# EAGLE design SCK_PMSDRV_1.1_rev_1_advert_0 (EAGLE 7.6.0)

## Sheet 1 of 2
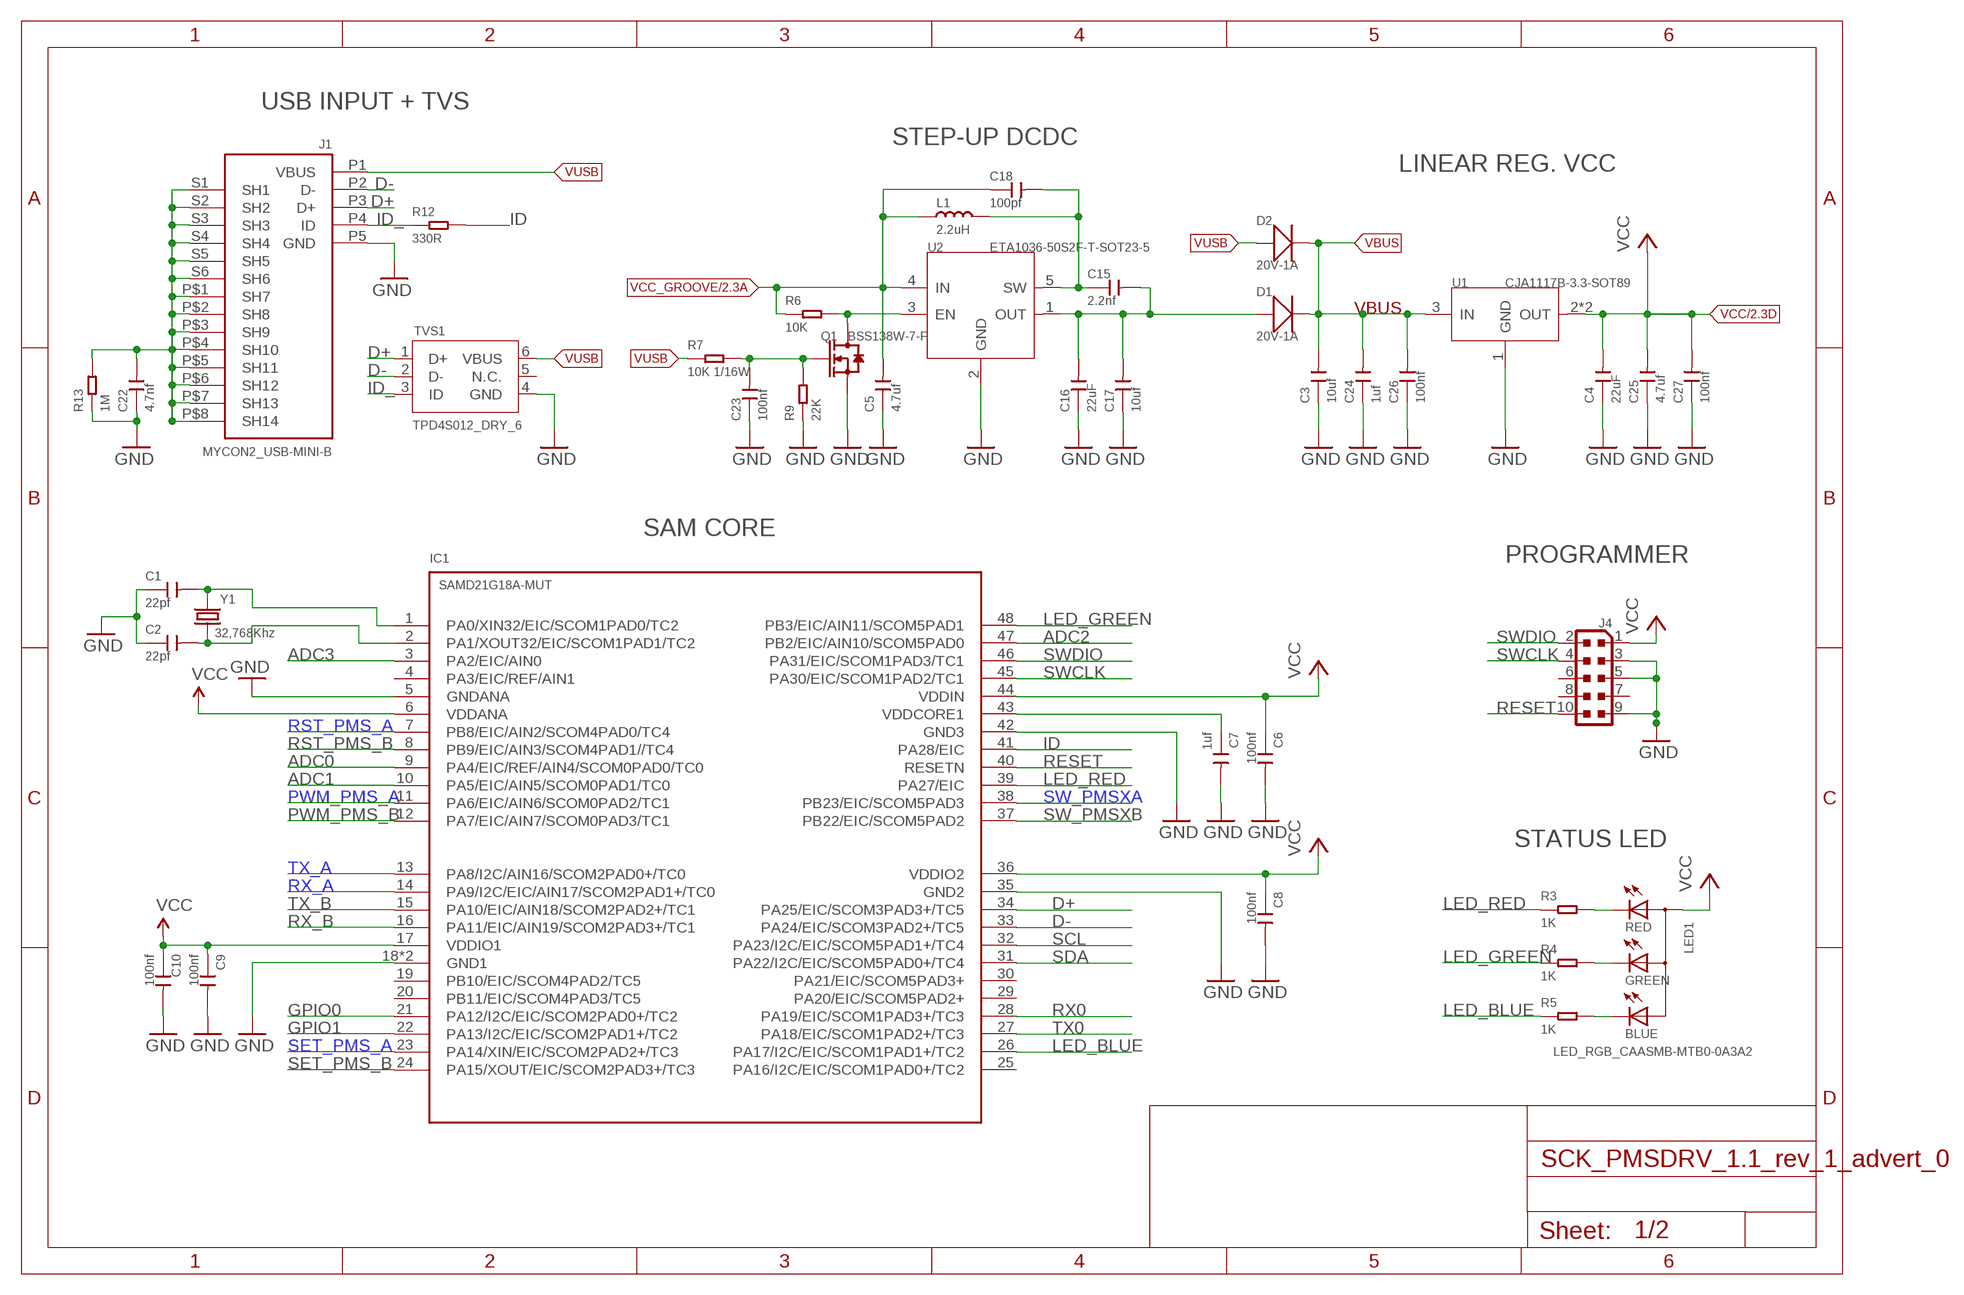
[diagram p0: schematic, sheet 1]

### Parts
C1  22pf  CERAMIC-22PF-50V-5%-NPO(0402)  [C0402]
C2  22pf  CERAMIC-22PF-50V-5%-NPO(0402)  [C0402]
C3  10uf  CERAMIC-10UF-25V-10%-X5R(1206)  [C1206]
C4  22uF  CERAMIC-22UF-16V-10%-X7R(1206)  [C1206]
C5  4.7uf  CERAMIC-4.7UF-25V-10%-X5R(0805)  [C0805]
C6  100nf  CERAMIC-100NF-50V-10%-X7R(0603)  [C0603]
C7  1uf  CERAMIC-1UF-25V-10%-X7R(0603)  [C0603]
C8  100nf  CERAMIC-100NF-50V-10%-X7R(0603)  [C0603]
C9  100nf  CERAMIC-100NF-50V-10%-X7R(0603)  [C0603]
C10  100nf  CERAMIC-100NF-50V-10%-X7R(0603)  [C0603]
C15  2.2nf  CERAMIC-2.2NF-50V-10%-X7R(0402)  [C0402]
C16  22uF  CERAMIC-22UF-16V-10%-X7R(1206)  [C1206]
C17  10uf  CERAMIC-10UF-25V-10%-X5R(1206)  [C1206]
C18  100pf  CERAMIC-100PF-50V-5%-NPO(0603)  [C0603]
C22  4.7nf  CERAMIC-4.7NF-50V-10%-X7R(0603)  [C0603]
C23  100nf  CERAMIC-100NF-50V-10%-X7R(0603)  [C0603]
C24  1uf  CERAMIC-1UF-25V-10%-X7R(0805)  [C0805]
C25  4.7uf  CERAMIC-4.7UF-25V-10%-X5R(0805)  [C0805]
C26  100nf  CERAMIC-100NF-50V-10%-X7R(0805)  [C0805]
C27  100nf  CERAMIC-100NF-50V-10%-X7R(0805)  [C0805]
D1  20V-1A  SMD-DIODE-SCHOTTKY-20V-1A(SOD-123)  [SOD-123]
D2  20V-1A  SMD-DIODE-SCHOTTKY-20V-1A(SOD-123)  [SOD-123]
IC1  SAMD21G18A-MUT  HANGAR_SAMD21G18A-MUT  [HANGAR_QFN48-7X7]
J1  MYCON2_USB-MINI-B  HANGAR_MYCON2_USB-MINI-B  [HANGAR_CON2_USB_MICRO_B_AT]
J4  HANGAR_PINHEAD_PINHD-2X5SMD  [HANGAR_2X05_SMD_1.27MM]
L1  2.2uH  SMD-INDUCTOR-10UH-20%-2.35A(2P-5X5X4MM)  [L5040S]
LED1  LED_RGB_CAASMB-MTB0-0A3A2  HANGAR_LED_RGB_CAASMB-MTB0-0A3A2  [HANGAR_P-LCC-4]
Q1  BSS138W-7-F  SMD-MOSFET-N-CH-50V-200MA-BSS138W-7-F(SOT-23)  [SOT-23]
R3  1K  SMD-RES-1K-5%-1/16W(0402)  [R0402]
R4  1K  SMD-RES-1K-5%-1/16W(0402)  [R0402]
R5  1K  SMD-RES-1K-5%-1/16W(0402)  [R0402]
R6  10K  SMD-RES-10K-1%-1/10W(0603)  [R0603]
R7  10K 1/16W  SMD-RES-10K-1%-1/16W(0402)  [R0402]
R9  22K  SMD-RES-22K-5%-1/10W(0603)  [R0603]
R12  330R  SMD-RES-330R-1%-1/10W(0603)  [R0603]
R13  1M  SMD-RES-1M-1%-1/10W(0603)  [R0603]
TVS1  TPD4S012_DRY_6  [DRY6]
U1  CJA1117B-3.3-SOT89  PMIC-CJA1117B-3.3(SOT-89)  [SOT-89]
U2  ETA1036-50S2F-T-SOT23-5  PMIC-ETA1036-50S2F-T(SOT23-5)  [SOT-23-5]
Y1  32,768Khz  0213_ABS07-32.768KHZ-T  [RESONATOR_EPSON_FC_145]

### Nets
ADC0: IC1.9(PA4/EIC/REF/AIN4/SCOM0PAD0/TC0) ; also sheet 2
ADC1: IC1.10(PA5/EIC/AIN5/SCOM0PAD1/TC0) ; also sheet 2
ADC2: IC1.47(PB2/EIC/AIN10/SCOM5PAD0) ; also sheet 2
ADC3: IC1.3(PA2/EIC/AIN0) ; also sheet 2
D+: IC1.34(PA25/EIC/SCOM3PAD3+/TC5) J1.P3(D+) TVS1.1(D+)
D-: IC1.33(PA24/EIC/SCOM3PAD2+/TC5) J1.P2(D-) TVS1.2(D-)
GND: C1.1 C2.1 C3.1 C4.1 C5.1 C6.2 C7.2 C8.2 C9.2 C10.2 C16.1 C17.1 C22.1 C23.1 C24.1 C25.1 C26.1 C27.1 IC1.5(GNDANA) IC1.18(GND1) IC1.35(GND2) IC1.42(GND3) IC1.TP(GND1) J1.P5(GND) J4.3 J4.5 J4.9 Q1.2(S) R9.1 R13.1 TVS1.4(GND) U1.1(GND) U2.2(GND) ; also sheet 2
GPIO0: IC1.21(PA12/I2C/EIC/SCOM2PAD0+/TC2) ; also sheet 2
GPIO1: IC1.22(PA13/I2C/EIC/SCOM2PAD1+/TC2) ; also sheet 2
ID: IC1.41(PA28/EIC) R12.2
ID_: J1.P4(ID) R12.1 TVS1.3(ID)
LED_BLUE: IC1.26(PA17/I2C/EIC/SCOM1PAD1+/TC2) R5.1
LED_GREEN: IC1.48(PB3/EIC/AIN11/SCOM5PAD1) R4.1
LED_RED: IC1.39(PA27/EIC) R3.1
N$1: LED1.4(RED) R3.2
N$2: LED1.3(GREEN) R4.2
N$3: LED1.2(BLUE) R5.2
N$4: C7.1 IC1.43(VDDCORE1)
N$6: Q1.3(D) R6.2 U2.3(EN)
N$7: C23.2 Q1.1(G) R7.2 R9.2
N$8: C15.1 C18.2 L1.2 U2.5(SW)
PA00_XIN32: C1.2 IC1.1(PA0/XIN32/EIC/SCOM1PAD0/TC2) Y1.P$2
PA01_XOUT32: C2.2 IC1.2(PA1/XOUT32/EIC/SCOM1PAD1/TC2) Y1.P$1
PWM_PMS_A: IC1.11(PA6/EIC/AIN6/SCOM0PAD2/TC1) ; also sheet 2
PWM_PMS_B: IC1.12(PA7/EIC/AIN7/SCOM0PAD3/TC1) ; also sheet 2
RESET: IC1.40(RESETN) J4.10
RST_PMS_A: IC1.7(PB8/EIC/AIN2/SCOM4PAD0/TC4) ; also sheet 2
RST_PMS_B: IC1.8(PB9/EIC/AIN3/SCOM4PAD1//TC4) ; also sheet 2
RX0: IC1.28(PA19/EIC/SCOM1PAD3+/TC3) ; also sheet 2
RX_A: IC1.14(PA9/I2C/EIC/AIN17/SCOM2PAD1+/TC0) ; also sheet 2
RX_B: IC1.16(PA11/EIC/AIN19/SCOM2PAD3+/TC1) ; also sheet 2
SCL: IC1.32(PA23/I2C/EIC/SCOM5PAD1+/TC4) ; also sheet 2
SDA: IC1.31(PA22/I2C/EIC/SCOM5PAD0+/TC4) ; also sheet 2
SET_PMS_A: IC1.23(PA14/XIN/EIC/SCOM2PAD2+/TC3) ; also sheet 2
SET_PMS_B: IC1.24(PA15/XOUT/EIC/SCOM2PAD3+/TC3) ; also sheet 2
SHIELD: C22.2 J1.P$1(SH7) J1.P$2(SH8) J1.P$3(SH9) J1.P$4(SH10) J1.P$5(SH11) J1.P$6(SH12) J1.P$7(SH13) J1.P$8(SH14) J1.S1(SH1) J1.S2(SH2) J1.S3(SH3) J1.S4(SH4) J1.S5(SH5) J1.S6(SH6) R13.2
SW_PMSXA: IC1.38(PB23/EIC/SCOM5PAD3) ; also sheet 2
SW_PMSXB: IC1.37(PB22/EIC/SCOM5PAD2) ; also sheet 2
SWCLK: IC1.45(PA30/EIC/SCOM1PAD2/TC1) J4.4
SWDIO: IC1.46(PA31/EIC/SCOM1PAD3/TC1) J4.2
TX0: IC1.27(PA18/EIC/SCOM1PAD2+/TC3) ; also sheet 2
TX_A: IC1.13(PA8/I2C/AIN16/SCOM2PAD0+/TC0) ; also sheet 2
TX_B: IC1.15(PA10/EIC/AIN18/SCOM2PAD2+/TC1) ; also sheet 2
VBUS: C3.2 C24.2 C26.2 D1.- D2.- U1.3(IN) ; also sheet 2
VCC [usbvcc]: C4.2 C6.1 C8.1 C9.1 C10.1 C25.2 C27.2 IC1.6(VDDANA) IC1.17(VDDIO1) IC1.36(VDDIO2) IC1.44(VDDIN) J4.1 LED1.1(A) U1.2(OUT) U1.4(OUT) ; also sheet 2
VCC_GROOVE: C5.2 C18.1 L1.1 R6.1 U2.4(IN) ; also sheet 2
VO_DCDC: C15.2 C16.2 C17.2 D1.+ U2.1(OUT)
VUSB: D2.+ J1.P1(VBUS) R7.1 TVS1.6(VBUS)
Unconnected: IC1.4(PA3/EIC/REF/AIN1) IC1.19(PB10/EIC/SCOM4PAD2/TC5) IC1.20(PB11/EIC/SCOM4PAD3/TC5) IC1.25(PA16/I2C/EIC/SCOM1PAD0+/TC2) IC1.29(PA20/EIC/SCOM5PAD2+) IC1.30(PA21/EIC/SCOM5PAD3+) J4.6 J4.7 J4.8 TVS1.5(N.C.)

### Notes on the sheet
- USB INPUT + TVS
- STEP-UP DCDC
- LINEAR REG. VCC
- SAM CORE
- PROGRAMMER
- STATUS LED

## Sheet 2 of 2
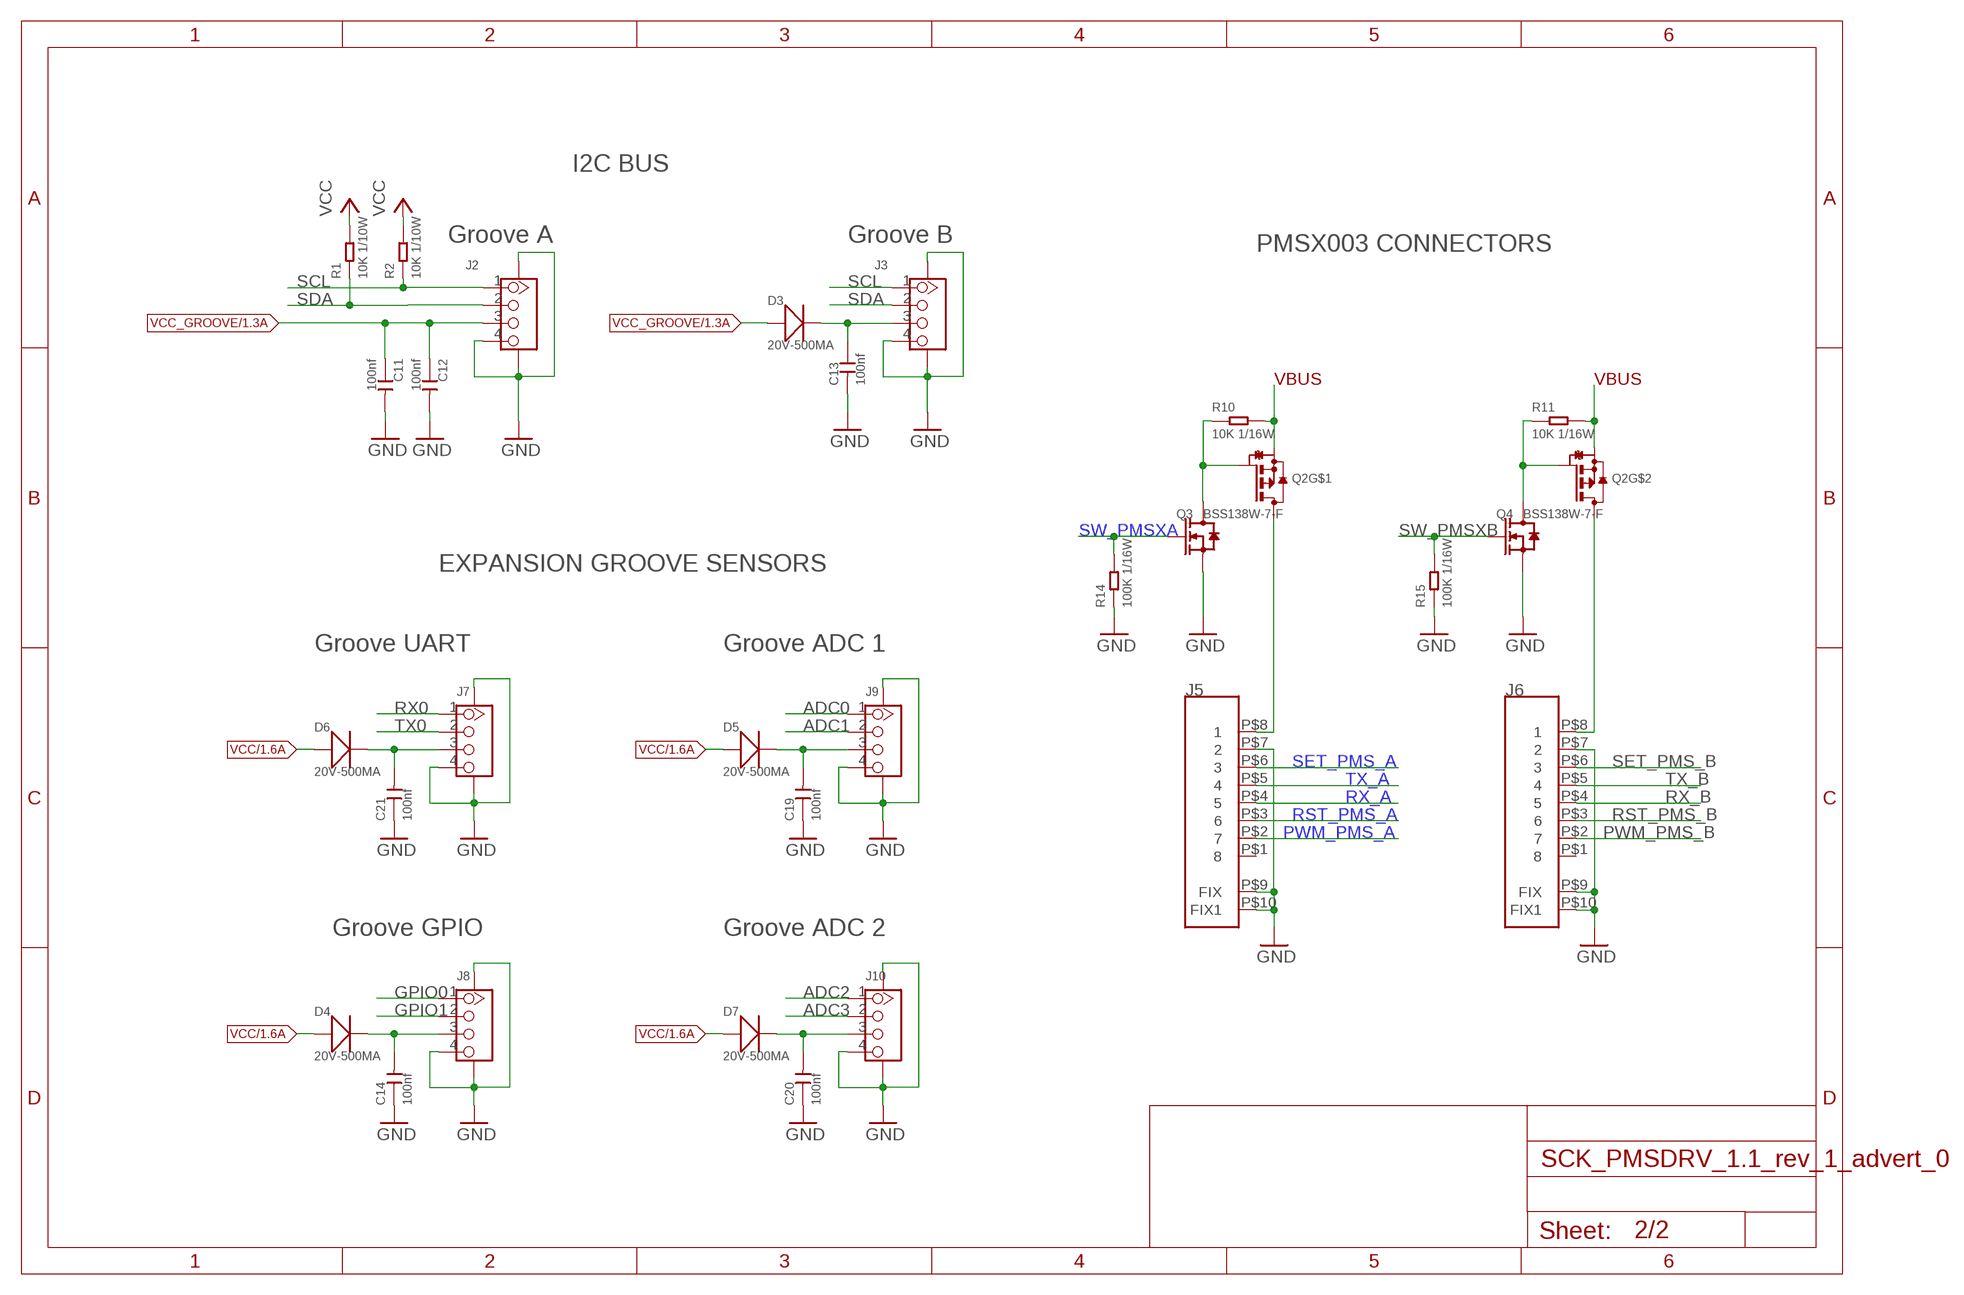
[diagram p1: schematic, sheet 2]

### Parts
C11  100nf  CERAMIC-100NF-50V-10%-X7R(0603)  [C0603]
C12  100nf  CERAMIC-100NF-50V-10%-X7R(0603)  [C0603]
C13  100nf  CERAMIC-100NF-50V-10%-X7R(0603)  [C0603]
C14  100nf  CERAMIC-100NF-50V-10%-X7R(0603)  [C0603]
C19  100nf  CERAMIC-100NF-50V-10%-X7R(0603)  [C0603]
C20  100nf  CERAMIC-100NF-50V-10%-X7R(0603)  [C0603]
C21  100nf  CERAMIC-100NF-50V-10%-X7R(0603)  [C0603]
D3  20V-500MA  SMD-DIODE-SCHOTTKY-20V-500MA(SOD-123)P  [SOD-123]
D4  20V-500MA  SMD-DIODE-SCHOTTKY-20V-500MA(SOD-123)P  [SOD-123]
D5  20V-500MA  SMD-DIODE-SCHOTTKY-20V-500MA(SOD-123)P  [SOD-123]
D6  20V-500MA  SMD-DIODE-SCHOTTKY-20V-500MA(SOD-123)P  [SOD-123]
D7  20V-500MA  SMD-DIODE-SCHOTTKY-20V-500MA(SOD-123)P  [SOD-123]
J2  CONNECTOR-NEW_GROVE-CONNECTOR-SMD90D  [CONNECTOR-NEW_HW4-SMD-2.0-90D]
J3  CONNECTOR-NEW_GROVE-CONNECTOR-SMD90D  [CONNECTOR-NEW_HW4-SMD-2.0-90D]
J5  MOLEX_53398-0871_8PIN  [MOLEX_PICOBLADE_8PIN]
J6  MOLEX_53398-0871_8PIN  [MOLEX_PICOBLADE_8PIN]
J7  CONNECTOR-NEW_GROVE-CONNECTOR-SMD90D  [CONNECTOR-NEW_HW4-SMD-2.0-90D]
J8  CONNECTOR-NEW_GROVE-CONNECTOR-SMD90D  [CONNECTOR-NEW_HW4-SMD-2.0-90D]
J9  CONNECTOR-NEW_GROVE-CONNECTOR-SMD90D  [CONNECTOR-NEW_HW4-SMD-2.0-90D]
J10  CONNECTOR-NEW_GROVE-CONNECTOR-SMD90D  [CONNECTOR-NEW_HW4-SMD-2.0-90D]
Q2  MOSFETP_BOTH  [HANGAR_POWERPAKSC70-6L]
Q3  BSS138W-7-F  SMD-MOSFET-N-CH-50V-200MA-BSS138W-7-F(SOT-23)  [SOT-23]
Q4  BSS138W-7-F  SMD-MOSFET-N-CH-50V-200MA-BSS138W-7-F(SOT-23)  [SOT-23]
R1  10K 1/10W  SMD-RES-10K-5%-1/10W(0603)  [R0603]
R2  10K 1/10W  SMD-RES-10K-5%-1/10W(0603)  [R0603]
R10  10K 1/16W  SMD-RES-10K-1%-1/16W(0402)  [R0402]
R11  10K 1/16W  SMD-RES-10K-1%-1/16W(0402)  [R0402]
R14  100K 1/16W  SMD-RES-100K-5%-1/16W(0402)  [R0402]
R15  100K 1/16W  SMD-RES-100K-5%-1/16W(0402)  [R0402]

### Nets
ADC0: J9.1 ; also sheet 1
ADC1: J9.2 ; also sheet 1
ADC2: J10.1 ; also sheet 1
ADC3: J10.2 ; also sheet 1
GND: C11.2 C12.2 C13.2 C14.1 C19.1 C20.1 C21.1 J2.4 J2.SS1 J2.SS2 J3.4 J3.SS1 J3.SS2 J5.P$7 J5.P$9(FIX) J5.P$10(FIX1) J6.P$7 J6.P$9(FIX) J6.P$10(FIX1) J7.4 J7.SS1 J7.SS2 J8.4 J8.SS1 J8.SS2 J9.4 J9.SS1 J9.SS2 J10.4 J10.SS1 J10.SS2 Q3.2(S) Q4.2(S) R14.1 R15.1 ; also sheet 1
GPIO0: J8.1 ; also sheet 1
GPIO1: J8.2 ; also sheet 1
N$9: J5.P$8 Q2.6(D) Q2.TP1(D)
N$10: J6.P$8 Q2.3(D) Q2.TP2(D)
N$12: C14.2 D4.- J8.3
N$13: C19.2 D5.- J9.3
N$14: C21.2 D6.- J7.3
N$15: C20.2 D7.- J10.3
N$16: C13.1 D3.- J3.3
PWM_PMS_A: J5.P$2 ; also sheet 1
PWM_PMS_B: J6.P$2 ; also sheet 1
RST_PMS_A: J5.P$3 ; also sheet 1
RST_PMS_B: J6.P$3 ; also sheet 1
RX0: J7.1 ; also sheet 1
RX_A: J5.P$4 ; also sheet 1
RX_B: J6.P$4 ; also sheet 1
SCL: J2.1 J3.1 R2.1 ; also sheet 1
SDA: J2.2 J3.2 R1.1 ; also sheet 1
SET_PMS_A: J5.P$6 ; also sheet 1
SET_PMS_B: J6.P$6 ; also sheet 1
SW_PMSXA: Q3.1(G) R14.2 ; also sheet 1
SW_PMSXA_NEG: Q2.2(G) Q3.3(D) R10.1
SW_PMSXB: Q4.1(G) R15.2 ; also sheet 1
SW_PMSXB_NEG: Q2.5(G) Q4.3(D) R11.1
TX0: J7.2 ; also sheet 1
TX_A: J5.P$5 ; also sheet 1
TX_B: J6.P$5 ; also sheet 1
VBUS: Q2.1(S) Q2.4(S) R10.2 R11.2 ; also sheet 1
VCC [usbvcc]: D4.+ D5.+ D6.+ D7.+ R1.2 R2.2 ; also sheet 1
VCC_GROOVE: C11.1 C12.1 D3.+ J2.3 ; also sheet 1
Unconnected: J5.P$1 J6.P$1

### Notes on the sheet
- I2C BUS
- Groove A | Groove B
- PMSX003 CONNECTORS
- EXPANSION GROOVE SENSORS
- Groove UART | Groove ADC 1
- Groove GPIO | Groove ADC 2

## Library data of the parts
C1 C2 = Seeed-Capacitor:CERAMIC-22PF-50V-5%-NPO(0402): 302010018; MPN: CC0402JRNPO9BN220
C3 C17 = Seeed-Capacitor:CERAMIC-10UF-25V-10%-X5R(1206): 302010181; MPN: CC1206KKX5R8BB106
C4 C16 = Seeed-Capacitor:CERAMIC-22UF-16V-10%-X7R(1206): 302010182
C5 C25 = Seeed-Capacitor:CERAMIC-4.7UF-25V-10%-X5R(0805): 302010146; MPN: CC0805KKX5R8BB475
C6 C8-C14 C19-C21 C23 = Seeed-Capacitor:CERAMIC-100NF-50V-10%-X7R(0603): 302010138; MPN: CC0603KRX7R9BB104
C7 = Seeed-Capacitor:CERAMIC-1UF-25V-10%-X7R(0603): 302010139; MPN: CC0603KRX7R8BB105
C15 = Seeed-Capacitor:CERAMIC-2.2NF-50V-10%-X7R(0402): 302010022; MPN: CC0402KRX7R9BB222
C18 = Seeed-Capacitor:CERAMIC-100PF-50V-5%-NPO(0603): 302010076; MPN: CC0603JRNPO9BN101
C22 = Seeed-Capacitor:CERAMIC-4.7NF-50V-10%-X7R(0603): 302010144; MPN: CC0603KRX7R9BB472
C24 = Seeed-Capacitor:CERAMIC-1UF-25V-10%-X7R(0805): 302010179; MPN: CC0805KKX7R8BB105
C26 C27 = Seeed-Capacitor:CERAMIC-100NF-50V-10%-X7R(0805): 302010165; MPN: CC0805KRX7R9BB104
D1 D2 = Seeed-OPL-Diode:SMD-DIODE-SCHOTTKY-20V-1A(SOD-123): 304020034; MPN: B5819W
D3-D7 = Seeed-Diode:SMD-DIODE-SCHOTTKY-20V-500MA(SOD-123)P: 304020028; MPN: MBR0520LT1G
IC1 = SCK_BASE_BOARD_v1.6:HANGAR_SAMD21G18A-: Atmel D21 32bit ARM Cortex-M0 microcontroller - 48 PIN TQFP 256KB flash memory + 32KB SRAM
J1 = SCK_BASE_BOARD_v1.6:HANGAR_MYCON2_USB-MINI-B
J2 J3 J7-J10 = SCK_BASE_BOARD_v1.6:CONNECTOR-NEW_GROVE-CONNECTOR-SMD: 4P-SMD-2.0:320110030;4P-SMD-2.0-90D:320110032
J4 = SCK_BASE_BOARD_v1.6:HANGAR_PINHEAD_PINHD-2X5: PIN HEADER
J5 J6 = SCK_BASE_BOARD_v1.6:MOLEX_53398-0871_8PIN
L1 = Seeed-Inductor:SMD-INDUCTOR-10UH-20%-2.35A(2P-5X5X4MM): 303010147
LED1 = SCK_BASE_BOARD_v1.6:HANGAR_LED_RGB_CA: PLCC-4 RGB LED
Q1 Q3 Q4 = Seeed-Transistor:SMD-MOSFET-N-CH-50V-200MA-BSS138W-7-F(SOT-23): 305030000; MPN: BSS138W-7-F
Q2 = SCK_BASE_BOARD_v1.6:MOSFETP_BOTH
R1 R2 = Seeed-Resistor:SMD-RES-10K-5%-1/10W(0603): 301010293; MPN: RC0603JR-0710KL
R3-R5 = Seeed-Resistor:SMD-RES-1K-5%-1/16W(0402): 301010006; MPN: RC0402JR-071KL
R6 = Seeed-Resistor:SMD-RES-10K-1%-1/10W(0603): 301010299; MPN: RC0603FR-0710KL
R7 R10 R11 = Seeed-Resistor:SMD-RES-10K-1%-1/16W(0402): 301010047; MPN: RC0402FR-0710KL
R9 = Seeed-Resistor:SMD-RES-22K-5%-1/10W(0603): 301010132; MPN: RC0603JR-0722KL
R12 = Seeed-Resistor:SMD-RES-330R-1%-1/10W(0603): 301010300; MPN: RC0603FR-07330RL
R13 = Seeed-Resistor:SMD-RES-1M-1%-1/10W(0603): 301010151; MPN: RC0603FR-071ML
R14 R15 = Seeed-Resistor:SMD-RES-100K-5%-1/16W(0402): 301010033; MPN: RC0402JR-07100KL
TVS1 = fabhack:TPD4S012_DRY_6
U1 = Seeed-IC:PMIC-CJA1117B-3.3(SOT-89): 310030095; MPN: CJA1117B-3.3
U2 = Seeed-IC:PMIC-ETA1036-50S2F-T(SOT23-5): 310030153; MPN: ETA1036-50S2F-T
Y1 = Cristalli:0213_ABS07-32.768KHZ-T: 32,768KHz - SMD; MONTHLY_USAGE: _____; PART_NUMBER: ABS07-32.768KHZ-T; PRICE: _____; SUPPLIER: _____; TYPE: Cristalli; VALUE: 32,768Khz_SMD

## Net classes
0 Default: width 0.203 mm
1 power: width 1 mm, drill 0.6 mm, clearance 0.203 mm
2 gnd: width 0.254 mm, drill 0.6 mm, clearance 0.203 mm
3 usbvcc: width 0.254 mm, drill 0.6 mm, clearance 0.203 mm
4 aref: width 0.254 mm, drill 0.6 mm, clearance 0.203 mm

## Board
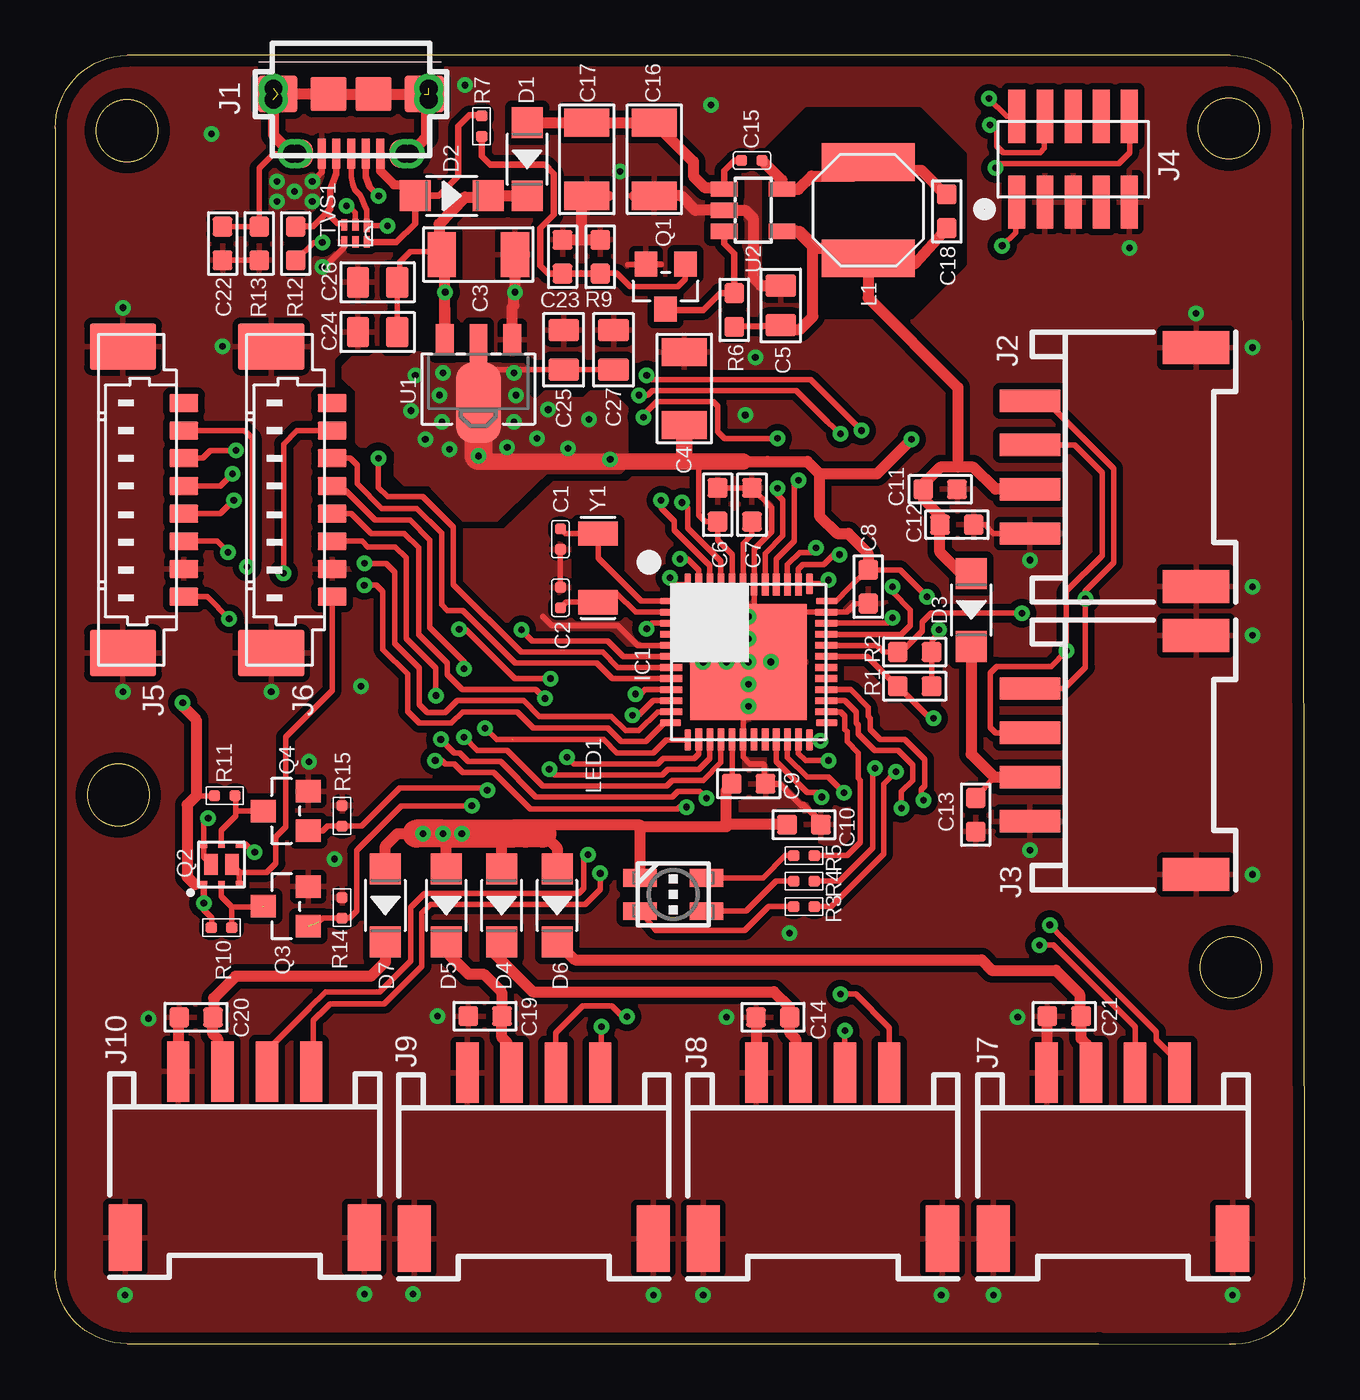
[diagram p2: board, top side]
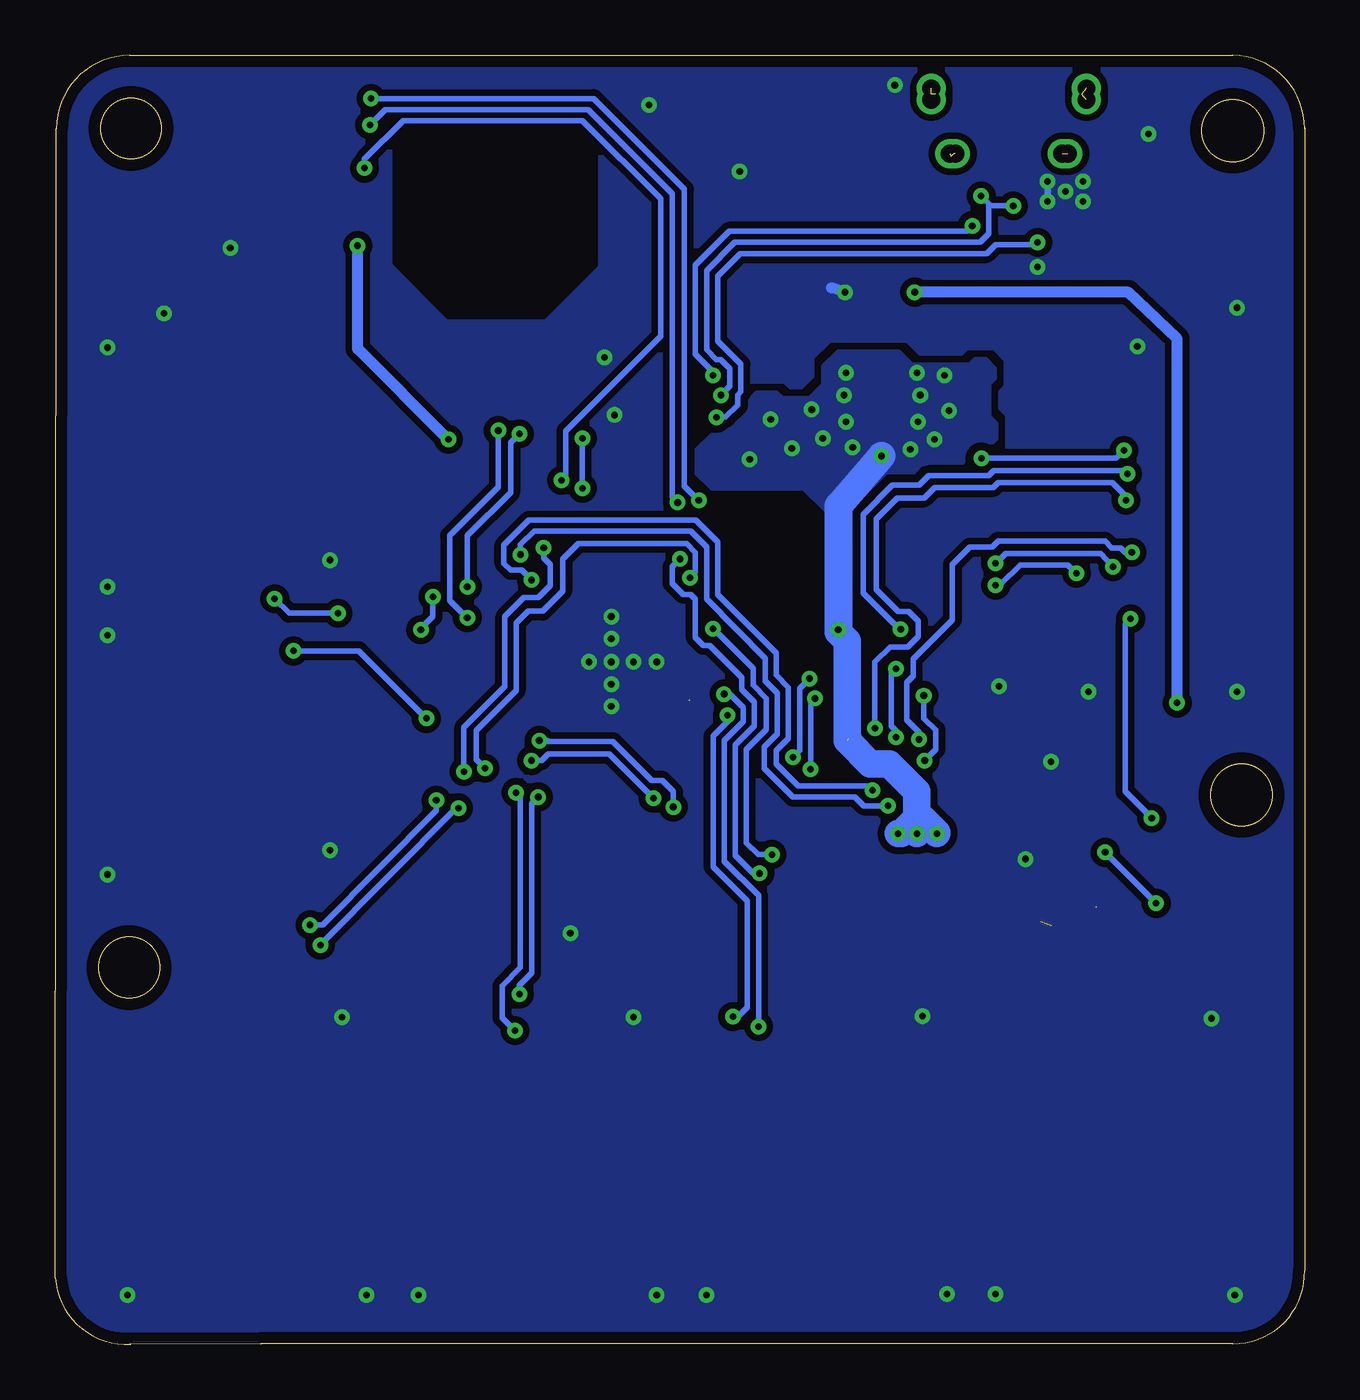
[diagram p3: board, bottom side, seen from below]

Size 56.4 x 58.21 mm. Coordinates in mm from the lower left corner, seen from the top.
Outline: 53,0 arc90 56.4,3.01 56.35,54.91 arc90 53.05,58.21 3.24,58.21 arc90 0,54.91
Outline: 0.9,0.98 arc45 3.24,0.02 47.11,0.02 arc90 47.12,0.02 53.03,0
Outline: 0.9,0.98 arc-45 0,3.32 0,54.94
Outline: circle at 53.07,17.01 radius 1.38
Outline: circle at 52.98,54.91 radius 1.38
Outline: circle at 3.24,54.81 radius 1.4
Outline: circle at 2.85,24.81 radius 1.4
Copper layers (1*16): Top 0.035mm / dielectric 1.5mm / Bottom 0.035mm
Design rules "default *": minimum track width 0.2mm, minimum drill 0.3mm, track to track 0.2mm, track to pad 0.2mm, pad to pad 0.2mm, via to via 0.2mm, smd to smd 0.2mm, copper to edge 20mil, drill to drill 0.6mm, minimum pad ring 10mil, minimum via ring 0.2mm, stop-mask expansion 2mil, vias tented up to drill 24mil, thermal gap 10mil

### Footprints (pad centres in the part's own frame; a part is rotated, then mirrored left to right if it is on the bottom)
C0402 = smd 0.5 x 0.5: 1 0,0.463; 2 0,-0.463
C1206 = smd 1.27 x 2.032: 1 -1.651,0; 2 1.651,0
C0805 = smd 1.397 x 1.016: 1 0,0.889; 2 0,-0.889
C0603 = smd 0.889 x 0.889: 1 0,0.762; 2 0,-0.762
SOD-123 = smd 1.397 x 1.397: + -1.651,0; - 1.651,0
HANGAR_QFN48-7X7 = smd 0.95 x 0.3: 1 -3.525,2.75; 12 -3.525,-2.75; 25 3.525,-2.75; 36 3.525,2.75 | smd 1 x 0.3: 2 -3.5,2.25; 3 -3.5,1.75; 4 -3.5,1.25; 5 -3.5,0.75; 6 -3.5,0.25; 7 -3.5,-0.25; 8 -3.5,-0.75; 9 -3.5,-1.25; 10 -3.5,-1.75; 11 -3.5,-2.25; 26 3.5,-2.25; 27 3.5,-1.75; 28 3.5,-1.25; 29 3.5,-0.75; 30 3.5,-0.25; 31 3.5,0.25; 32 3.5,0.75; 33 3.5,1.25; 34 3.5,1.75; 35 3.5,2.25 | smd 0.3 x 0.95: 13 -2.75,-3.525; 24 2.75,-3.525; 37 2.75,3.525; 48 -2.75,3.525 | smd 0.3 x 1: 14 -2.25,-3.5; 15 -1.75,-3.5; 16 -1.25,-3.5; 17 -0.75,-3.5; 18 -0.25,-3.5; 19 0.25,-3.5; 20 0.75,-3.5; 21 1.25,-3.5; 22 1.75,-3.5; 23 2.25,-3.5; 38 2.25,3.5; 39 1.75,3.5; 40 1.25,3.5; 41 0.75,3.5; 42 0.25,3.5; 43 -0.25,3.5; 44 -0.75,3.5; 45 -1.25,3.5; 46 -1.75,3.5; 47 -2.25,3.5 | smd 5.25 x 5.25: TP 0,0
HANGAR_CON2_USB_MICRO_B_AT = smd 0.406 x 1.346: P1 -1.321,2.692; P2 -0.66,2.692; P3 0,2.692; P4 0.66,2.692; P5 1.321,2.692 | drill 0.8 pad 1.27: P$1 -2.666,2.692 | drill 0.8 pad 1.245: P$2 -2.412,2.692; P$7 2.412,2.692; P$8 2.666,2.692 | drill 0.8 pad 1.143: P$3 -3.505,-0.254; P$4 -3.505,0.254; P$5 3.505,0.254; P$6 3.505,-0.254 | smd 1.778 x 1.651: S1 -3.302,0; S2 3.302,0 | smd 1.524 x 1.27: S3 -2.489,2.692; S4 2.489,2.692 | smd 1.626 x 1.524: S5 -1.016,0; S6 1.016,0
CONNECTOR-NEW_HW4-SMD-2.0-90D = smd 1.01 x 2.74: 1 -3,-0.1; 2 -1,-0.1; 3 1,-0.1; 4 3,-0.1 | smd 1.5 x 3: SS1 -5.4,7.4; SS2 5.4,7.4
HANGAR_2X05_SMD_1.27MM = smd 0.76 x 2.4: 1 -2.54,-1.94; 2 -2.54,1.94; 3 -1.27,-1.94; 4 -1.27,1.94; 5 0,-1.94; 6 0,1.94; 7 1.27,-1.94; 8 1.27,1.94; 9 2.54,-1.94; 10 2.54,1.94
MOLEX_PICOBLADE_8PIN = smd 0.8 x 1.3: P$1 0,0; P$2 1.25,0; P$3 2.5,0; P$4 3.75,0; P$5 5,0; P$6 6.25,0; P$7 7.5,0; P$8 8.75,0 | smd 2.1 x 3: P$9 -2.55,-2.75; P$10 11.3,-2.75
L5040S = smd 4.2 x 1.7: 1 0,2.175; 2 0,-2.175
HANGAR_P-LCC-4 = smd 0.8 x 1.5: 1 -0.75,-1.5; 2 -0.75,1.5; 3 0.75,1.5; 4 0.75,-1.5
SOT-23 = smd 1.016 x 1.143: 1 -0.889,-1.016; 2 0.889,-1.016; 3 0,1.016
HANGAR_POWERPAKSC70-6L = smd 0.3 x 0.325: 1 -0.8,-0.912; 2 0,-0.912; 3 0.8,-0.912; 4 0.8,0.912; 5 0,0.912; 6 -0.8,0.912 | smd 0.613 x 0.95: TP1 -0.467,0; TP2 0.467,0
R0603 = smd 0.889 x 0.889: 1 0,0.762; 2 0,-0.762
R0402 = smd 0.5 x 0.5: 1 0,0.463; 2 0,-0.463
DRY6 = smd 0.559 x 0.305: 1 -0.356,0.508 | smd 0.508 x 0.305: 2 -0.381,0; 3 -0.381,-0.508; 4 0.381,-0.508; 5 0.381,0; 6 0.381,0.508
SOT-89 = smd 0.8 x 1.4: 1 -1.524,-1.905; 3 1.524,-1.905 | smd 0.8 x 1.9: 2 0,-1.651 | smd 2.032 x 3.65: 4 0,0.94
SOT-23-5 = smd 0.69 x 1.2: 1 -0.95,-1.3; 2 0,-1.3; 3 0.95,-1.3; 4 0.95,1.3; 5 -0.95,1.3
RESONATOR_EPSON_FC_145 = smd 1.1 x 1.8: P$1 -1.55,0; P$2 1.55,0

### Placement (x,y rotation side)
C1  22.8,36.36 180 top
C2  22.8,33.71 0 top
C3  19.1,49.21 180 top
C4  28.4,43.16 270 top
C5  32.75,46.91 0 top
C6  29.9,37.91 180 top
C7  31.45,37.91 180 top
C8  36.7,34.21 0 top
C9  31.3,25.31 90 top
C10  33.8,23.46 90 top
C11  39.95,38.61 90 top
C12  40.7,37.01 90 top
C13  41.55,23.91 0 top
C14  32.4,14.76 90 top
C15  31.45,53.46 270 top
C16  27.05,53.51 90 top
C17  24,53.51 90 top
C18  40.25,51.16 180 top
C19  19.4,14.81 90 top
C20  6.35,14.76 90 top
C21  45.55,14.81 90 top
C22  7.55,49.71 180 top
C23  22.9,49.11 0 top
C24  14.55,45.71 90 top
C25  22.95,44.91 0 top
C26  14.55,47.96 90 top
C27  25.2,44.91 0 top
D1  21.3,53.51 270 top
D2  17.9,51.86 0 top
D3  41.35,33.16 270 top
D4  20.15,19.81 270 top
D5  17.65,19.81 270 top
D6  22.65,19.81 270 top
D7  14.9,19.81 270 top
IC1  31.3,30.81 0 top
J1  13.35,56.46 180 top
J2  44.1,39.61 270 top
J3  44.1,26.61 270 top
J4  45.95,53.51 0 top
J5  5.8,42.51 270 top
J6  12.5,42.51 270 top
J7  47.75,12.16 180 top
J8  34.65,12.16 180 top
J9  21.6,12.16 180 top
J10  8.55,12.21 180 top
L1  36.7,51.21 180 top
LED1  27.9,20.31 270 top
Q1  27.55,47.76 180 top
Q2  7.5,21.66 0 top
Q3  10.4,19.78 90 top
Q4  10.4,24.08 90 top
R1  38.8,29.71 90 top
R2  38.8,31.26 90 top
R3  33.8,19.76 270 top
R4  33.8,20.91 270 top
R5  33.8,22.06 270 top
R6  30.65,46.71 180 top
R7  19.25,55.01 0 top
R9  24.6,49.11 0 top
R10  7.5,18.81 270 top
R11  7.65,24.76 270 top
R12  10.85,49.71 0 top
R13  9.2,49.71 180 top
R14  12.95,19.71 0 top
R15  12.95,23.86 0 top
TVS1  13.55,50.16 270 top
U1  19.1,43.46 180 top
U2  31.5,51.21 270 top
Y1  24.5,35.06 90 top

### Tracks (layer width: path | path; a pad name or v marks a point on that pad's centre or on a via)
ADC0  (via drill 0.3)
  Top 0.25: v24.65,14.35 24.65,12.31 J9.1 | IC1.9 26.6,29.56 26.45,29.36 v26.2,29.36
  Bottom 0.25: v24.65,14.35 24.65,20.26 26.2,21.81 26.2,27.26 25.35,28.11 25.35,28.76 25.95,29.36 v26.2,29.36
ADC1  (via drill 0.3)  (1 unrouted)
  Top 0.25: J9.2 22.6,14.06 23.81,15.27 25.12,15.27 25.6,14.8 v25.81,14.8 | 27.75,29.06 27,29.06 26.35,28.41 v26.05,28.41
  Bottom 0.25: v26.05,28.41 26.05,28.11 26.7,27.46 26.7,21.56 25.15,20.01 25.15,15.21 25.61,14.75 25.82,14.79 v25.81,14.8
ADC2  (via drill 0.3)
  Top 0.25: IC1.47 29.05,34.97 28.56,35.46 v28.2,35.46 | J10.1 11.65,12.41 11.65,14.62 11.94,14.91 11.94,14.9 12.4,15.36 14.85,15.36 16.55,17.06 16.55,19.47 16.94,19.86 23.92,19.86 24.6,20.54 v24.6,21.26
  Bottom 0.25: v24.6,21.26 24.9,21.26 25.7,22.06 25.7,27.06 24.85,27.91 24.85,29.01 25.4,29.56 25.4,30.11 26.85,31.56 27.15,31.56 27.5,31.91 27.5,33.65 27.71,33.86 28.05,33.86 28.55,34.36 28.55,35.11 v28.2,35.46
ADC3  (via drill 0.3)
  Top 0.25: J10.2 9.55,13.25 11.46,15.16 11.46,15.18 12.2,15.91 14.65,15.91 16.05,17.31 16.05,19.73 16.68,20.36 23.63,20.36 23.85,20.59 23.85,21.91 v24.05,22.11 | IC1.3 26.95,32.56 v26.7,32.31
  Bottom 0.25: v26.7,32.31 24.9,30.51 24.9,29.76 24.3,29.16 24.3,27.76 25.2,26.86 25.2,22.64 24.67,22.11 v24.05,22.11
D+  (via drill 0.3)
  Top 0.25: J1.P3 13.35,52.73 13.42,52.4 13.52,52.14 13.77,51.89 13.85,51.7 13.95,51.46 14.05,51.22 TVS1.1 v15,50.51 | v36.4,41.26 36.1,41.58 35.46,42.21 35.45,42.21 34.1,43.56 26.9,43.56 v26.7,43.76 | v37.8,32.81 37.55,32.56 IC1.34
  Bottom 0.25: v36.4,41.26 36.4,38.71 38.59,36.52 38.6,33.59 37.82,32.81 v37.8,32.81 | v15,50.51 15.25,50.26 25.98,50.26 27.5,48.74 27.5,44.71 26.7,43.91 v26.7,43.76
D-  (via drill 0.3)
  Top 0.25: v35.45,41.11 34.85,41.66 33.45,43.06 26.95,43.06 26.75,42.86 v26.35,42.86 | v37.8,34.21 37.8,33.96 38.6,33.16 38.6,32.46 38.2,32.06 IC1.33 | TVS1.2 13.55,51.11 13.25,51.41 v13.15,51.41
  Top 0.3: J1.P2 14.01,52.72 14.2,52.26 v14.6,51.86
  Bottom 0.25: 14.25,51.41 v13.15,51.41 | v35.45,41.11 35.85,40.71 35.85,38.46 37.8,36.51 v37.8,34.21 | 14.25,51.41 14.25,50.16 14.65,49.76 25.73,49.76 27,48.49 27,44.91 26.55,44.46 26.35,44.46 25.95,44.06 25.95,43.26 v26.35,42.86 | 14.25,51.41 14.25,51.51 v14.6,51.86
GND  (via drill 0.3)
  Top 0.25: C9.2 32.26,25.3 32,25.31 32,26.16 31.95,26.21 31.35,26.21 31.05,26.51 IC1.18 31.05,28.76 31.1,28.81 31.1,30.61 IC1.TP | C10.2 34.6,23.47 | C2.1 C1.1 | 31.55,31.06 IC1.42 31.55,35.91 32.35,36.71 32.35,37.77 C7.2 C6.2 | 31.55,31.06 33.55,33.06 IC1.35 35.73,33.06 36.1,33.44 C8.2 36.7,33.51 36.75,33.51 | 31.55,31.06 IC1.TP | IC1.TP 30.55,31.56 IC1.5 26.3,31.56 25.4,32.46 22.4,32.46 22,32.86 | Q1.2 27.35,48.78 27.35,48.76 25.85,48.76 | 24.4,49.91 24.75,49.87 24.74,49.87 | TVS1.4 13.04,49.55 12.2,48.71 v12.05,48.66 | 24.7,51.61 24,51.61 23.75,51.86 | 23.75,49.92 23.7,49.87 | C22.1 R13.1 | J2.4 42.35,36.61 41.95,37.01 C12.2
  Top 0.3: 34.6,23.47 34.6,23.56 33.8,24.36 33.65,24.36 32.7,25.31 C9.2 | J1.P5 12.03,52.94 v11.6,52.51
  Top 0.5: C5.1 31.86,47.8 31.5,48.16 31.5,50.86 31.15,51.21 U2.2 28.9,51.21 28.25,51.86 27.55,51.86 C16.1 26.15,51.86 | C20.1 5.55,14.72 J10.4 | C14.1 31.65,14.75 J8.4 | C21.1 44.75,14.77 J7.4 | 40.7,38.56 C11.2 | C17.1 24.95,51.86 | C23.1 23.7,49.87 R9.1 24.74,49.87 | 23.75,51.86 23.75,49.92 | C3.1 20.75,47.71 v20.75,47.51 20.7,47.66 20.7,46.91 20.62,46.84 U1.1
  Bottom 0.3: v11.6,52.51 v11.6,51.61
  Bottom 0.5: v20.75,47.51 21.35,47.71
  other vias: 31.3,32.86 31.3,29.81 30.3,30.81 44,35.41 53.15,2.21 48.5,49.51 25.5,52.96 51.5,46.56 54.05,32.01 54.05,45.01 54.05,34.21 10.8,52.06 16.15,2.26 40,2.21 29.25,2.21 42.35,2.21 13.95,2.26 27,2.21 54.05,21.21 3.15,2.21 4.2,14.71 17.25,14.81 30.3,14.76 43.45,14.76 44,22.31 31.6,44.56 3.05,29.46 9.75,29.46 3.05,46.81 7.55,45.06 10,51.61 10,52.51 31.3,30.81 31.3,31.86 29.25,30.81 32.3,30.81 31.3,28.81 7.05,54.66 29.6,55.96 11.45,26.31 13.8,29.71 12.6,21.91 31.15,41.96 18.5,56.86 33.15,18.56
  pour Bottom (isolate 0.3, rank 2): -0.5,-0.94 37.5,-1.29 57.4,-1.29 56.45,58.21 56.5,59.21 -0.4,59.21
  pour Top (isolate 0.3, rank 2): -0.5,-0.94 37.5,-1.04 57.25,-1.04 57.25,59.56 -0.3,59.36
GPIO0  (via drill 0.3)
  Top 0.25: IC1.21 32.55,26.31 33.95,24.91 34.4,24.91 v34.6,24.71 | v35.45,15.81 36.13,15.81 37.65,14.29 J8.1
  Bottom 0.25: v34.6,24.71 34.9,24.41 34.9,16.76 35.45,16.21 v35.45,15.81
GPIO1  (via drill 0.3)
  Top 0.25: IC1.22 33.05,26.51 33.95,25.61 34.9,25.61 v35.6,24.91 | v35.65,14.16 J8.2
  Bottom 0.25: v35.6,24.91 35.4,24.71 35.4,17.01 36.23,16.18 36.23,14.74 v35.65,14.16
ID  (via drill 0.3)
  Top 0.25: v32.6,40.91 32.6,40.96 32.56,40.9 30.21,40.9 29.9,41.21 29.9,42.36 29.7,42.56 27.16,42.56 26.55,41.95 v26.55,41.86 | R12.2 11.66,49.75 v12.05,49.76 | v32.6,38.66 32.59,38.36 32.85,38.12 32.85,36.51 32.05,35.71 IC1.41
  Bottom 0.25: v32.6,38.66 v32.6,40.91 | v12.05,49.76 12.15,49.66 13.95,49.66 14.35,49.26 25.47,49.26 26.5,48.24 26.5,45.31 25.45,44.26 25.45,43.01 25.6,42.86 25.6,42.41 26.15,41.86 v26.55,41.86
ID_
  Top 0.25: TVS1.3 12.97,50.61 12.75,50.61 12.35,51.01 12.35,51.16 12.4,51.19 12.32,51.19
  Top 0.3: J1.P4 12.69,52.85 12.55,52.51 12.4,52.15 12.4,51.26 12.32,51.19 11.95,50.81 11.64,50.5 R12.1
LED_BLUE
  Top 0.25: IC1.26 35.45,28.56 35.65,28.36 35.65,27.76 35.75,27.66 35.75,27.21 36.25,26.71 36.25,25.56 36.35,25.46 36.35,22.66 35.75,22.06 R5.1
LED_GREEN  (via drill 0.3)
  Top 0.25: IC1.48 28.52,34.31 28.05,34.31 v27.75,34.61 | R4.1 35.41,20.91 36.9,22.4 36.9,25.91 v37,26.01
  Bottom 0.25: v27.75,34.61 27.5,34.86 27.5,35.76 27.9,36.16 32.8,36.16 33.5,35.46 33.5,34.01 34.4,33.11 35.05,33.11 35.6,32.56 35.6,29.51 37.4,27.71 37.4,26.41 v37,26.01
LED_RED  (via drill 0.3)
  Top 0.25: IC1.39 33.05,35.21 33.6,35.76 34.15,35.76 v34.35,35.96 | R3.1 35.03,19.76 37.4,22.13 37.4,25.31 v37.95,25.86
  Bottom 0.25: v34.35,35.96 34.35,35.51 34.05,35.21 34.05,34.26 34.6,33.71 35.25,33.71 36.1,32.86 36.1,29.71 37.95,27.86 v37.95,25.86
N$1
  Top 0.25: LED1.4 27.11,18.69 31.12,18.68 32.2,19.76 R3.2
N$2
  Top 0.25: LED1.3 31.2,19.56 32.55,20.91 R4.2
N$3
  Top 0.25: LED1.2 31.95,21.06 32.95,22.06 R5.2
N$4
  Top 0.25: IC1.43 31.05,36.16 31.45,36.56 C7.1
N$5
  cutout Top (isolate 0.35, no thermals): 32.02,53.83 33.95,55.75 39.01,55.75 41.03,53.73 41.03,48.81 38.64,46.42 34.35,46.42 32.02,48.75
  cutout Bottom (isolate 0.35, no thermals): 32.02,53.91 33.86,55.74 39.84,55.74 41.06,54.52 41.06,48.84 38.64,46.41 34.37,46.41 32.02,48.75
N$6
  Top 0.3: U2.3 30.2,49.71 30.65,49.26 R6.2 30.01,47.47 29.25,46.71 28.12,46.71 Q1.3
  Top 0.406: U2.3
N$7
  Top 0.25: Q1.1 28.45,48.11 28.1,47.76 25.95,47.76 25.35,48.36 24.61,48.36 R9.2
  Top 0.3: Q1.1 | R7.2 19.25,53.65 19.64,53.26 22.11,53.26 22.5,52.87 22.5,51.01 21.9,50.41 21.9,48.71 22.26,48.35 C23.2 23.75,48.35 | R9.2 23.75,48.35 | 23.75,48.36 23.75,48.35
N$8
  Top 0.406: L1.2 36.7,53.01 | 40.19,51.91 C18.2
  Top 0.5: C15.1 32.8,52.57 U2.5 33.55,52.16 34.15,52.76 36.08,52.76 L1.2 | 36.7,53.01 39.1,53.01 40.19,51.91
N$9  (via drill 0.3)
  Top 0.25: Q2.TP1 6.7,21.99 Q2.6 6.7,23.56 v6.9,23.76 | v7.85,32.76 6.85,33.76 J5.P$8
  Bottom 0.25: v6.9,23.76 8.1,24.96 8.1,32.51 v7.85,32.76
N$10
  Top 0.25: 8.3,21.31 8.3,21.33 Q2.TP2 7.97,21.65 8.3,21.31 | 8.3,21.31 Q2.3 | 8.3,21.31 9.55,21.31 9.95,21.71 9.95,22.91 10.4,23.36 10.4,27.41 12.5,29.51 J6.P$8
N$12
  Top 0.5: J8.3 33.45,12.46 33.45,13.76 33.16,14.05 C14.2 33.15,14.77 33.15,15.2 32.44,15.91 21.55,15.91 19.8,17.66 D4.-
N$13
  Top 0.5: J9.3 20.4,12.46 20.4,13.61 20.16,13.85 C19.2 20.15,14.82 20.15,15.9 19.34,16.71 18.65,16.71 17.8,17.56 D5.-
N$14
  Top 0.5: J7.3 46.55,12.46 46.55,13.56 46.31,13.8 C21.2 46.25,14.87 46.25,15.81 45.17,16.88 42.28,16.88 42.25,16.91 41.82,17.36 23.45,17.36 22.2,18.61 D6.-
N$15
  Top 0.5: J10.3 7.35,12.51 7.35,13.76 7.11,14 C20.2 7.15,14.8 7.15,15.62 8.14,16.61 13.35,16.61 14.1,16.61 14.25,16.61 14.9,17.26 14.9,17.91 D7.-
N$16
  Top 0.25: C13.1 42.39,25.61
  Top 0.5: D3.- 41.35,26.65 42.39,25.61 J3.3
PA00_XIN32
  Top 0.25: IC1.1 26.45,33.56 24.5,35.51 Y1.P$2 23.01,36.61 C1.2
PA01_XOUT32
  Top 0.25: IC1.2 26.2,33.06 25.35,33.91 24.9,33.91 Y1.P$1 23.06,33.51 C2.2
PWM_PMS_A  (via drill 0.3)
  Top 0.25: IC1.11 27.2,28.56 26.35,27.71 25.75,27.71 25.11,28.35 21.86,28.35 21.15,29.06 18.14,29.06 17.61,28.53 16.79,28.53 16.43,28.89 16.43,30.54 15.32,31.65 15.32,34.88 14.95,35.25 v13.96,35.25 v13.95,35.26 | J5.P$2 8.55,41.26 8.89,40.92 8.89,35.35 v8.65,35.11
  Bottom 0.25: v13.95,35.26 13.5,35.71 9.2,35.71 v8.65,35.11
PWM_PMS_B  (via drill 0.3)
  Top 0.25: J6.P$2 10.9,41.26 10.3,40.66 v10.3,34.81 | IC1.12 27.5,28.06 26.65,27.21 25.55,27.21 24.93,27.83 21.58,27.83 20.85,28.56 18.39,28.56 17.87,28.05 16.43,28.05 15.9,28.58 15.9,30.27 14.79,31.38 14.79,33.98 14.49,34.28 v13.95,34.28
  Bottom 0.25: v13.95,34.28 13.92,34.3 13.73,34.3 12.82,35.19 10.69,35.2 v10.3,34.81
RESET  (via drill 0.3)
  Top 0.25: J4.10 48.5,53.81 48,53.31 42.7,53.31 42.51,53.12 v42.44,53.12 | v33.55,39.01 33.35,38.81 33.35,36.26 32.55,35.46 IC1.40
  Bottom 0.25: 32.6,55.26 29.07,51.74 29.07,45.52 33.35,41.25 33.35,39.21 v33.55,39.01 | 32.6,55.26 40.7,55.26 42.45,53.51 42.45,53.26 v42.44,53.12 | 32.6,55.26 32.61,55.27
RST_PMS_A  (via drill 0.3)
  Top 0.25: IC1.7 25.4,30.56 24.7,31.26 21.02,31.26 17.97,34.31 17.97,36.9 16.59,38.27 15,38.27 14.59,38.69 v14.59,40.01 | v8.15,40.36 7,40.36 6.65,40.01 J5.P$3
  Bottom 0.25: v14.59,40.01 8.5,40.01 v8.15,40.36
RST_PMS_B
  Top 0.25: IC1.8 25.15,30.06 24.44,30.77 20.76,30.77 18.4,33.13 17.7,33.13 17.44,33.4 17.44,36.63 16.32,37.74 14.73,37.74 13.62,38.86 13.62,39.71 13.3,40.02 12.51,40.02 J6.P$3
RX0  (via drill 0.3)
  Top 0.25: J7.1 50.75,12.71 49.71,13.75 49.71,14.11 45.53,18.29 v44.9,18.93 | IC1.28 35.9,29.56 36.7,28.76 36.7,28.36 36.8,28.26 36.8,27.76 37.25,27.31 38.35,27.31 39.25,26.41 39.25,25.21 39.1,25.06 39.1,24.66 v39.2,24.56
  Bottom 0.25: v44.9,18.93 44.33,18.93 39.2,24.11 v39.2,24.56
RX_A  (via drill 0.3)
  Top 0.25: IC1.14 29.05,26.66 28.85,26.46 27.45,26.46 27.2,26.21 23.4,26.21 v23.1,26.51 | v22.35,30.06 20.75,30.06 18.53,32.29 v18.23,32.29 | J5.P$4 7.45,38.76 v8,39.31
  Bottom 0.25: v8,39.31 8.14,39.45 14.03,39.45 14.26,39.23 16.96,39.23 17.38,38.8 18.6,38.8 19.93,37.48 19.93,33.93 18.29,32.29 v18.23,32.29 | v23.1,26.51 22.8,26.81 22.8,29.61 v22.35,30.06
RX_B  (via drill 0.3)
  Top 0.25: J6.P$4 12.8,38.76 13,38.56 13.1,38.56 14.45,37.21 16.02,37.21 16.9,36.33 16.9,32.36 18.45,30.81 v18.45,30.51 | IC1.16 30.05,26.26 29.25,25.46 27.85,25.46 27.6,25.21 22,25.21 20.4,26.81 19.05,26.81 v18.45,27.41
  Bottom 0.25: v18.45,30.51 18.65,30.31 18.65,27.91 18.45,27.71 v18.45,27.41
SCL  (via drill 0.3)
  Top 0.25: v43.64,33.01 39.55,33.01 39.15,32.61 39.15,32.21 38.2,31.26 R2.1 37.4,31.26 37.1,31.56 IC1.32 | J2.1 44.72,42.61 47.78,39.55 47.78,35.3 46.5,34.01 v46.5,33.66 46.5,30.57 45.55,29.61 J3.1
  Bottom 0.25: v43.64,33.01 45.85,33.01 v46.5,33.66
SDA  (via drill 0.3)
  Top 0.25: IC1.31 36.65,31.06 38,29.71 R1.1 38.05,29.7 38.45,29.31 39.5,28.26 v39.65,28.26 | J2.2 46.02,40.61 47.26,39.36 47.26,35.63 45.65,34.01 v45.65,31.31 44.95,30.61 42.5,30.61 42.2,30.31 42.2,27.86 42.45,27.61 J3.2
  Bottom 0.25: v45.65,31.31 42.7,31.31 v39.65,28.26
SET_PMS_A  (via drill 0.3)
  Top 0.25: IC1.23 33.55,26.68 33.87,26.36 v34.9,26.36 | v29.4,24.66 29.1,24.96 28.1,24.96 27.85,24.71 21.7,24.71 20.1,26.31 18.65,26.31 18.25,26.71 18,26.71 v17.4,27.31 | v7.8,35.76 7.3,36.26 J5.P$6
  Bottom 0.25: v34.9,26.36 34.45,26.36 34.15,26.66 31.4,26.66 v29.4,24.66 | v7.8,35.76 8.1,35.76 8.3,35.96 8.7,35.96 9,36.26 13.83,36.26 14.1,35.99 15.12,35.99 15.9,35.21 15.9,32.72 17.68,30.94 17.68,30.17 17.96,29.89 17.96,28.18 17.4,27.62 v17.4,27.31
SET_PMS_B  (via drill 0.3)
  Top 0.25: IC1.24 34.08,27.26 v34.55,27.26 | J6.P$6 13.85,36.26 14.1,36.01 15.35,36.01 15.85,35.52 15.85,31.86 17.17,30.54 17.17,29.31 v17.19,29.29 17.23,29.32 | v28.5,24.26 28.2,24.26 28.1,24.16 21.45,24.16 19.8,25.81 18.4,25.81 18,26.21 17.6,26.21 17.45,26.36 v17.15,26.36
  Bottom 0.25: v34.55,27.26 34.2,27.26 34.15,27.21 31.22,27.21 29.47,25.46 29,25.46 28.5,24.96 v28.5,24.26 | v17.19,29.29 17.19,28.26 16.65,27.74 16.65,26.86 v17.15,26.36
SHIELD  (9 unrouted)
  Top 0.25: C22.2 R13.2 9.2,53.11 9.85,53.76 J1.P$8
  Top 0.5: J1.P$1 | J1.S2 J1.S6 J1.S5 16.85,56.46 J1.P$4 16.75,56.15 16.75,54.51 15.95,53.66 16.35,53.66 | J1.P$5 9.85,54.61 J1.P$8
SW_PMSXA  (via drill 0.3)  (1 unrouted)
  Top 0.25: IC1.38 33.55,35.01 33.75,35.21 34.7,35.21 35.15,35.66 v35.4,35.66 | v18.8,24.31 15.62,24.31 13.6,22.29 13.6,19.56 13.29,19.25 R14.2 12.84,19.26 12.1,19.26 11.9,19.06
  Bottom 0.25: v35.4,35.66 35.4,36.1 34.78,36.72 27.71,36.72 27,36.01 27,33.66 24.35,30.96 24.35,29.96 23.8,29.41 23.8,27.56 24.4,26.96 24.4,26.01 23.1,24.71 20.3,24.71 19.9,24.31 v18.8,24.31
SW_PMSXA_NEG  (1 unrouted)
  Top 0.25: Q2.2 7.5,20.21 7.96,19.75 | 7.96,19.75 R10.1 | 9.41,19.75 7.96,19.75
SW_PMSXB  (via drill 0.3)
  Top 0.25: IC1.37 34.08,34.36 34.75,34.36 v34.9,34.51 | v19.5,25.01 19.38,25.13 15.69,25.13 15.55,25.12 13.84,23.41 12.91,23.41 R15.2 12.89,23.41 12.3,23.41 12.08,23.19 Q4.1
  Bottom 0.25: v34.9,34.51 35.35,34.96 35.85,34.96 36.15,35.26 36.15,36.08 35.02,37.21 27.48,37.21 26.5,36.23 26.5,33.86 23.85,31.21 23.85,30.21 23.3,29.66 23.3,27.36 23.85,26.81 23.85,26.21 22.85,25.21 19.7,25.21 v19.5,25.01
SW_PMSXB_NEG
  Top 0.25: R11.1 8.15,24.72 8.15,24.06 | 8.15,24.06 8.15,23.86 7.5,23.21 Q2.5 | Q4.3 8.17,24.08 8.15,24.06
SWCLK  (via drill 0.3)
  Top 0.25: IC1.45 30.05,35.36 28.55,36.86 28.55,37.76 v28.3,38.01 | J4.4 44.65,55.42 44.65,54.01 44.46,53.82 42.79,53.82 42.5,54.11 42.5,54.81 42.25,55.06 v42.2,55.06
  Bottom 0.25: v28.3,38.01 28.54,38.27 28.54,51.95 32.35,55.76 41.5,55.76 v42.2,55.06
SWDIO  (via drill 0.3)
  Top 0.25: IC1.46 29.55,35.16 27.95,36.76 27.95,37.17 27.35,37.77 v27.35,38.11 | J4.2 42.96,55.45 v42.15,56.26
  Bottom 0.25: v27.35,38.11 28,38.76 28,52.16 32.1,56.26 v42.15,56.26
TX0  (via drill 0.3)
  Top 0.25: IC1.27 35.65,29.06 36.15,28.56 36.15,28.06 36.25,27.96 36.25,27.56 37,26.81 38.05,26.81 38.7,26.16 38.7,25.46 38.2,24.96 v38.2,24.21 | J7.2 48.75,14.33 45.05,18.03 44.49,18.03 v44.44,18.02
  Bottom 0.25: v38.2,24.21 38.3,24.21 v44.44,18.02
TX_A  (via drill 0.3)
  Top 0.25: IC1.13 27.57,27.29 27,26.71 25.35,26.71 24.76,27.3 19.94,27.3 v19.4,27.81 | J5.P$5 7.45,37.51 v8.06,38.12
  Bottom 0.25: v19.4,27.81 19.4,30.8 18.71,31.49 17.91,31.49 17.44,31.97 17.44,32.66 17.86,33.08 18.34,33.08 19.34,34.09 19.34,37.27 18.39,38.22 17.17,38.22 16.7,38.7 14.04,38.7 13.83,38.91 8.69,38.91 8.06,38.27 v8.06,38.12
TX_B  (via drill 0.3)
  Top 0.25: J6.P$5 13.35,37.51 14.25,36.61 15.76,36.61 16.4,35.97 16.4,32.06 17.7,30.76 17.7,30.24 18.38,29.56 21.7,29.56 v22.1,29.16 | IC1.15 29.55,26.46 29.05,25.96 27.65,25.96 27.4,25.71 22.55,25.71 v22.3,25.96
  Bottom 0.25: v22.3,25.96 22.3,28.96 v22.1,29.16
VBUS  (via drill 0.3)
  Top 0.25: R11.2 6.35,24.76 | R10.2 7.05,18.82 7.05,19.26 6.7,19.61 v6.7,19.91 | Q2.4 8.31,22.56 | 9,22.16 v9,22.21 | C24.2 C26.2 | 17.33,49.33 16.02,49.33 15.55,48.86 15.55,48.07 | v17.6,47.51 17.58,47.49 17.58,47.21
  Top 0.3: 6.31,20.75 Q2.1 v6.7,19.91 | 8.31,22.56 8.6,22.56 9,22.16
  Top 0.5: 17.57,46.81 U1.3 17.58,47.21 17.58,49.08 C3.2 17.33,49.33 17.33,50.59 18.5,51.81 20.05,51.81 20,51.71 20,51.81 20.05,51.86 | 21.25,51.81 D1.- 20.05,51.86 | D2.- 20.05,51.86 | 6.31,20.75 5.95,21.11 5.95,24.36 6.35,24.76 6.35,28.21 5.75,28.81 v5.75,28.96 | 15.55,48.07 C26.2
  Bottom 0.3: v9,22.21 v6.7,19.91
  Bottom 0.5: v5.75,28.96 5.75,45.41 7.95,47.51 v17.6,47.51
VCC  (via drill 0.3)  (1 unrouted)
  Top 0.25: IC1.17 30.55,25.41 30.3,25.16 30.3,25.07 C9.1 30.55,25.32 | IC1.44 30.55,35.66 29.9,36.31 C6.1 29.34,37.15 29.05,37.44 29.05,39.86 | IC1.6 25.65,31.06 24.95,31.76 21.53,31.76 21.05,32.24 v21.05,32.26 | IC1.36 35.25,33.56 35.85,34.16 36.66,34.97 C8.1 38.14,34.97 v39.35,33.76 | C27.2 C25.2 19.11,44.02 | v39.9,32.26 39.9,32.11 39.6,31.81 39.6,31.3 R2.2 R1.2 | J4.1 43.35,51.51 43.35,50.21 v42.75,49.61 | 26.39,23.45 26.4,23.45 26.4,23.36
  Top 0.3: 30.3,25.05 C9.1 | 32.14,39.87 32.15,39.86 | U1.2 19.1,44.01 U1.4
  Top 0.5: 30.3,23.36 30.3,25.05 | D7.+ 14.9,22.51 15.45,23.06 16.3,23.06 | v17.5,23.06 21.23,23.06 | D6.+ 22.65,22.41 22,23.06 19.6,23.11 20.15,23.11 D4.+ | D5.+ 17.65,23.01 17.8,23.06 | 31.05,39.86 32.15,39.86 33.95,39.86 34.5,39.31 | LED1.1 26.4,23.29 26.39,23.45 20.74,23.45 20.65,23.06 | C10.1 30.4,23.46 30.3,23.36 | 30.3,23.36 26.4,23.36 26.3,23.46 | C8.1 36.7,35.71 35.8,36.61 35.3,36.61 34.5,37.41 34.5,39.31 | v38.65,40.86 37.1,39.31 34.5,39.31 | 19.11,44.02 19.1,44.01
  Top 0.75: 31.05,39.86 29.05,39.86 28.35,39.86 | 28.35,39.86 19.15,39.86 v19.1,40.11 | C4.2 28.4,39.91 28.35,39.86
  Top 1.27: v17.5,23.06 17.8,23.06 | v17.5,23.06 16.3,23.06 | v17.5,23.06 20.65,23.06 21.23,23.06 22,23.06 | U1.4 v19.1,40.11
  Bottom 0.25: v39.9,32.26 39.9,32.31 39.35,32.86 v39.35,33.76
  Bottom 0.5: v38.65,40.86 42.75,44.96 v42.75,49.61
  Bottom 1.25: v21.05,32.26 21.05,32.16 20.65,31.76 20.65,27.41 20.6,27.36 | 20.65,27.26 19.6,26.21 18.75,26.21 17.5,24.96 17.5,24.01 | 17.5,24.01 17.5,23.76 | 17.5,23.76 v17.5,23.06 | v16.6,23.06 16.6,23.11 17.5,24.01 | v18.35,23.06 18.2,23.06 17.5,23.76
  Bottom 1.27: v19.1,40.11 21.05,37.86 v21.05,32.26
  other vias: 17.5,43.86 17.35,42.86 17.45,41.66 20.7,43.86 20.8,42.86 20.7,41.66 22.25,42.21 16.05,42.16 16.25,43.76 20.4,40.51 17.8,40.41 16.7,40.86 21.75,40.91 24.1,41.76 23.15,40.46 25.05,39.96
  pour Top (isolate 0.35, no thermals): 21.05,44.21 16.95,44.21 16.45,44.71 16.25,44.71 16.05,44.51 14.8,44.51 14.65,44.66 14.4,44.66 14.25,44.51 13.45,44.51 13.05,44.11 13.05,43.66 13.65,43.06 13.65,40.76 13.8,40.61 15.1,40.61 15.41,40.32 15.39,39.27 15.8,38.86 16.9,38.86 18.4,37.26 19.9,37.26 22.15,39.41 25.45,39.41 25.75,39.71 25.75,42.26 25.05,42.96 24.2,42.96 23.9,42.66 23.3,42.66 23,42.96 22.15,42.96 21.8,42.61 21.5,42.61 21.3,42.81 21.3,43.96
  pour Bottom (isolate 0.35, no thermals): 17.75,44.21 15.1,44.21 14.85,44.46 14.4,44.46 14,44.06 14,43.66 14.25,43.41 14.25,41.86 13.95,41.56 13.95,40.91 14.25,40.61 14.95,40.61 15.5,39.76 17.3,39.76 17.65,39.41 18.9,39.41 20.65,37.66 21.6,37.66 22.6,38.66 26.75,38.66 27.5,39.41 27.5,40.31 26.75,41.06 26.25,41.06 25.1,42.21 25.1,42.57 24.71,42.96 23.85,42.96 23.59,42.7 22.31,42.7 21.7,43.31 21.7,44.17 21.06,44.81 18.35,44.81
VCC_GROOVE
  Top 0.3: R6.1 30.81,45.96 30.55,45.96 31.94,45.97 C5.2
  Top 0.406: 36.23,49.51 L1.1 36.94,48.8 | U2.4
  Top 0.5: 36.23,49.51 34.35,49.51 33.6,50.26 U2.4 33.5,50.26 34.2,49.56 34.2,46.41 33.6,45.81 33.06,45.81 C5.2 | 38.8,48.8 36.94,48.8 | C18.1 38.8,48.8 | 38.8,48.8 36.7,48.76 36.7,47.26 40.75,43.21 40.75,39.61 | D3.+ 40.9,34.81 39.94,35.77 C12.1 39.94,37.42 39.2,38.16 C11.1 39.19,38.85 39.95,39.61 40.75,39.61 | J2.3 42.45,38.61 41.45,39.61 40.75,39.61
VO_DCDC
  Top 0.3: C15.2 30.66,53.46 30.2,53 U2.1
  Top 0.5: U2.1 30.15,52.21 29.35,52.21 28.8,52.76 28.8,53.41 C16.2 C17.2 21.6,55.16 D1.+
VUSB
  Top 0.3: TVS1.6 14.08,49.76 15.4,49.76 16.25,50.61 D2.+ 17.3,51.86 18.2,52.76 18.2,55.01 18.69,55.5 19.24,55.5 R7.1
  Top 0.4: J1.P1 14.67,52.99 15.3,52.36 15.75,52.36 D2.+

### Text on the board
200bmp: D:/Proyects/IAAC/PCBs/PMSDRIVR/SCK_PMSDRV_1.0/silk_screen/PM_BOARD-02_copia.bmp
201bmp: D:/Proyects/IAAC/PCBs/PMSDRIVR/SCK_PMSDRV_1.1/silk_screen/PM_BOARD-01 - copia v1.1 - advert.bmp
210bmp: SCL | SDA | VCC | I2C INPUT | GND | SCL | SDA | VCC | I2C OUTPUT | GND | GND | VCC | GND | VCC | ADC1 | VCC | GND | VCC | TX0 | RX0 | ADC3 | ADC2 | ADC0 | GND | GPIO1 | GPIO0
